| IBIS file stm32h563_573_ufbga201-smps.ibs
[IBIS ver] 4.2
[File name] stm32h563_573_ufbga201-smps.ibs
[File Rev] 1.1
[Date] 07-05-2024
[Source] Data Created at STMicroelectronics
[Notes]  File originated from ELDO simulations.
[Disclaimer]  This information is for modeling purpose only and is
   not guaranteed. The information is subject to change without
   notice.
[Copyright] Copyright 2024 STMicroelectronics Inc.
|   Component stm32h563_573_ufbga201-smps
[Component] stm32h563_573_ufbga201-smps
[Manufacturer] STMicroelectronics
[Package]
| variable   typ   min   max
R_pkg  0  NA  NA
L_pkg  0  NA  NA
C_pkg  0  NA  NA
[Pin]   signal_name   model_name
A1  PI7  io8_ft_i3c_spi
A2  PI5  io8_ft_i3c_spi
A3  VCAP  nc
A4  PB9  io8_ft_i3c_spi
A5  BOOT0  vpphv
A6  PB5  io8_ft_i3c_spi
A7  PG15  io8_ft_i3c_spi
A8  PG14  io8_ft_i3c_spi
A9  PG10  io8_ft_i3c_spi
A10  PD7  io8_ft_i3c_spi
A11  PD5  io8_ft_i3c_spi
A12  PD3  io8_ft_i3c_spi
A13  PD1  io8_ft_i3c_spi
A14  PI3  io8_ft_i3c_spi
A15  PI1  io8_ft_i3c_spi
B1  VBAT  power
B2  PE3  io8_ft_i3c_spi
B3  PI4  io8_ft_i3c_spi
B4  PE1  io8_ft_i3c_spi
B5  PB8  io8_ft_i3c_spi
B6  PB6  io8_ft_i3c_spi
B7  PB3  io8_ft_i3c_spi
B8  PG12  io8_ft_i3c_spi
B9  PG9  io8_ft_i3c_spi
B10  PD6  io8_ft_i3c_spi
B11  PD4  io8_ft_i3c_spi
B12  PD0  io8_ft_i3c_spi
B13  PA14  io8_ft_i3c_spi
B14  PI2  io8_ft_i3c_spi
B15  PH13  io8_ft_i3c_spi
C1  VSS  gnd
C2  PE6  io8_ft_i3c_spi
C3  PE4  io8_ft_i3c_spi
C4  PI6  io8_ft_i3c_spi
C5  PE0  io8_ft_i3c_spi
C6  PB7  io8_ft_i3c_spi
C7  PB4  io8_ft_i3c_spi
C8  PG13  io8_ft_i3c_spi
C9  PG11  io8_ft_i3c_spi
C10  PD2  io8_ft_i3c_spi
C11  PC12  io8_ft_i3c_spi
C12  PC11  io8_ft_i3c_spi
C13  PA15  io8_ft_i3c_spi
C14  PH15  io8_ft_i3c_spi
C15  PA12  io8usb_ft_i3c_spi_phy
D1  PC15-OSC32_OUT  io8_ft_i3c_spi
D2  PC14-OSC32_IN  io8_ft_i3c_spi
D3  PE5  io8_ft_i3c_spi
D4  PE2  io8_ft_i3c_spi
D5  VDD  power
D6  VSS  gnd
D7  VDDIO2  power
D8  VDD  power
D9  VSS  gnd
D10  VDD  power
D11  VSS  gnd
D12  PC10  io8_ft_i3c_spi
D13  PH14  io8_ft_i3c_spi
D14  VSS  gnd
D15  PA11  io8usb_ft_i3c_spi_phy
E1  PI9  io8_ft_i3c_spi
E2  PI8  io8_ft_i3c_spi
E3  PC13  io8_ft_i3c_spi
E4  VDD  power
E12  VDD  power
E13  PA13  io8_ft_i3c_spi
E14  PA10  io8_ft_i3c_spi
E15  PA9  io8_ft_i3c_spi
F1  PF1  io8_ft_i3c_spi
F2  PF0  io8_ft_i3c_spi
F3  PI11  io8_ft_i3c_spi
F4  PI10  io8_ft_i3c_spi
F6  VSS  gnd
F7  VSS  gnd
F8  VSS  gnd
F9  VSS  gnd
F10  VSS  gnd
F12  VDD33USB  power
F13  PC9  io8_ft_i3c_spi
F14  PC8  io8_ft_i3c_spi
F15  PA8  io8_ft_i3c_spi
G1  PF4  io8_ft_i3c_spi
G2  PF3  io8_ft_i3c_spi
G3  PF2  io8_ft_i3c_spi
G4  VSS  gnd
G6  VSS  gnd
G7  VSS  gnd
G8  VSS  gnd
G9  VSS  gnd
G10  VSS  gnd
G12  VSS  gnd
G13  PC7  io8_ft_i3c_spi
G14  PC6  io8_ft_i3c_spi
G15  PG8  io8_ft_i3c_spi
H1  PF6  io8_ft_i3c_spi
H2  PF8  io8_ft_i3c_spi
H3  PF5  io8_ft_i3c_spi
H4  VDD  power
H6  VSS  gnd
H7  VSS  gnd
H8  VSS  gnd
H9  VSS  gnd
H10  VSS  gnd
H12  VSS  gnd
H13  PG7  io8_ft_i3c_spi
H14  PG3  io8_ft_i3c_spi
H15  PG5  io8_ft_i3c_spi
J1  PH0-OSC_IN  io8_ft_i3c_spi
J2  PH1-OSC_OUT  io8_ft_i3c_spi
J3  PF9  io8_ft_i3c_spi
J4  PF10  io8_ft_i3c_spi
J6  VSS  gnd
J7  VSS  gnd
J8  VSS  gnd
J9  VSS  gnd
J10  VSS  gnd
J12  VDD  power
J13  PD15  io8_ft_i3c_spi
J14  PG6  io8_ft_i3c_spi
J15  PG4  io8_ft_i3c_spi
K1  VSS  gnd
K2  PF7  io8_ft_i3c_spi
K3  NRST  ioreset_ft_v33
K4  PC2  io8_ft_spi
K6  VSS  gnd
K7  VSS  gnd
K8  VSS  gnd
K9  VSS  gnd
K10  VSS  gnd
K12  PD10  io8_ft_i3c_spi
K13  PD14  io8_ft_i3c_spi
K14  PD12  io8_ft_i3c_spi
K15  PG2  io8_ft_i3c_spi
L1  PC0  io8_ft_spi
L2  PC1  io8_ft_spi
L3  PA1  io8_ft_spi_tamp
L4  VDD  power
L12  PB12  io8_ft_i3c_spi
L13  PD9  io8_ft_i3c_spi
L14  PD11  io8_ft_i3c_spi
L15  PD13  io8_ft_i3c_spi
M1  VDDA  nc
M2  VSSA  nc
M3  PA2  io8_ft_spi
M4  VSS  gnd
M5  PA4  io8_ft_spi
M6  VDD  power
M7  VSS  gnd
M8  VDD  power
M9  VSS  gnd
M10  PB10  io8_ft_i3c_spi
M11  VDD  power
M12  PH9  io8_ft_i3c_spi
M13  PH12  io8_ft_i3c_spi
M14  PB15  io8_ft_spi
M15  PD8  io8_ft_i3c_spi
N1  VREFP  nc
N2  VREFM  nc
N3  PC3  io8_ft_spi
N4  PC4  io8_ft_spi
N5  PA3  io8_ft_spi
N6  PB1  io8_ft_spi
N7  PF12  io8_ft_spi
N8  PF15  io8_ft_i3c_spi
N9  PE9  io8_ft_i3c_spi
N10  PE14  io8_ft_i3c_spi
N11  PE15  io8_ft_i3c_spi
N12  PB11  io8_ft_i3c_spi
N13  PH8  io8_ft_i3c_spi
N14  PH10  io8_ft_i3c_spi
|N15  PB14  io8usb_ft_pd
N15  PB14  nc
P1  PH5  io8_ft_i3c_spi
P2  PA0  io8_ft_spi
P3  PH3  io8_ft_i3c_spi
P4  PC5  io8_ft_spi
P5  PA6  io8_ft_spi
P6  PB2  io8_ft_i3c_spi
P7  PF13  io8_ft_spi
P8  PG1  io8_ft_i3c_spi
P9  PE8  io8_ft_i3c_spi
P10  PE11  io8_ft_i3c_spi
P11  PE13  io8_ft_i3c_spi
P12  VSSSMPS  nc
P13  PH6  io8_ft_i3c_spi
P14  PH7  io8_ft_i3c_spi
P15  PH11  io8_ft_i3c_spi
R1  PH4  io8_ft_i3c_spi
R2  PH2  io8_ft_i3c_spi
R3  PA5  io8_ft_spi
R4  PA7  io8_ft_spi
R5  PB0  io8_ft_spi
R6  PF11  io8_ft_spi
R7  PF14  io8_ft_spi
R8  PG0  io8_ft_i3c_spi
R9  PE7  io8_ft_i3c_spi
R10  PE10  io8_ft_i3c_spi
R11  PE12  io8_ft_i3c_spi
R12  VLXSMPS  nc
R13  VDDSMPS  nc
R14  VCAP  nc
|R15  PB13  io8usb_ft_pd
R15  PB13  nc
[Package Model]   484-ufbga-10x10-201-smps-221014
[Pin Mapping]   pulldown_ref   pullup_ref   | Comment
A1  gndio  vddiom
A2  gndio  vddiom
A3  nc  nc
A4  gndio  vddiom  | Depending on IO usage
| A4  gndio  vddmmc  | Depending on IO usage
A5  gndio  vddiom  | Depending on IO usage
| A5  gndio  vddmmc  | Depending on IO usage
A6  gndio  vddiom  | Depending on IO usage
| A6  gndio  vddmmc  | Depending on IO usage
A7  gndio  vddiom  | Depending on IO usage
| A7  gndio  vddmmc  | Depending on IO usage
A8  gndio  vddiom  | Depending on IO usage
| A8  gndio  vddmmc  | Depending on IO usage
A9  gndio  vddiom  | Depending on IO usage
| A9  gndio  vddmmc  | Depending on IO usage
A10  gndio  vddiom  | Depending on IO usage
| A10  gndio  vddmmc  | Depending on IO usage
A11  gndio  vddiom
A12  gndio  vddiom
A13  gndio  vddiom
A14  gndio  vddiom
A15  gndio  vddiom
B1  nc  vsw
B2  gndio  vddiom
B3  gndio  vddiom
B4  gndio  vddiom  | Depending on IO usage
| B4  gndio  vddmmc  | Depending on IO usage
B5  gndio  vddiom  | Depending on IO usage
| B5  gndio  vddmmc  | Depending on IO usage
B6  gndio  vddiom  | Depending on IO usage
| B6  gndio  vddmmc  | Depending on IO usage
B7  gndio  vddiom  | Depending on IO usage
| B7  gndio  vddmmc  | Depending on IO usage
B8  gndio  vddiom  | Depending on IO usage
| B8  gndio  vddmmc  | Depending on IO usage
B9  gndio  vddiom  | Depending on IO usage
| B9  gndio  vddmmc  | Depending on IO usage
B10  gndio  vddiom  | Depending on IO usage
| B10  gndio  vddmmc  | Depending on IO usage
B11  gndio  vddiom
B12  gndio  vddiom
B13  gndio  vddiom
B14  gndio  vddiom
B15  gndio  vddiom
C1  gndio  nc
C2  gndio  vddiom
C3  gndio  vddiom
C4  gndio  vddiom
C5  gndio  vddiom  | Depending on IO usage
| C5  gndio  vddmmc  | Depending on IO usage
C6  gndio  vddiom  | Depending on IO usage
| C6  gndio  vddmmc  | Depending on IO usage
C7  gndio  vddiom  | Depending on IO usage
| C7  gndio  vddmmc  | Depending on IO usage
C8  gndio  vddiom  | Depending on IO usage
| C8  gndio  vddmmc  | Depending on IO usage
C9  gndio  vddiom  | Depending on IO usage
| C9  gndio  vddmmc  | Depending on IO usage
C10  gndio  vddiom
C11  gndio  vddiom
C12  gndio  vddiom
C13  gndio  vddiom
C14  gndio  vddiom
C15  gndio  vddiom  | Depending on IO usage
| C15  gndio  vddusb  | Depending on IO usage
D1  gndio  vddiom  | Depending on IO usage
| D1  gndio  vsw  | Depending on IO usage
D2  gndio  vddiom  | Depending on IO usage
| D2  gndio  vsw  | Depending on IO usage
D3  gndio  vddiom
D4  gndio  vddiom
D5  nc  vddiom
D6  gndio  nc
D7  nc  vddmmc
D8  nc  vddiom
D9  gndio  nc
D10  nc  vddiom
D11  gndio  nc
D12  gndio  vddiom
D13  gndio  vddiom
D14  gndio  nc
D15  gndio  vddiom  | Depending on IO usage
| D15  gndio  vddusb  | Depending on IO usage
E1  gndio  vddiom
E2  gndio  vddiom  | Depending on IO usage
| E2  gndio  vsw  | Depending on IO usage
E3  gndio  vddiom  | Depending on IO usage
| E3  gndio  vsw  | Depending on IO usage
E4  nc  vddiom
E12  nc  vddiom
E13  gndio  vddiom  | Depending on IO usage
| E13  gndio  vddusb  | Depending on IO usage
E14  gndio  vddiom  | Depending on IO usage
| E14  gndio  vddusb  | Depending on IO usage
E15  gndio  vddiom  | Depending on IO usage
| E15  gndio  vddusb  | Depending on IO usage
F1  gndio  vddiom
F2  gndio  vddiom
F3  gndio  vddiom
F4  gndio  vddiom
F6  gndio  nc
F7  gndio  nc
F8  gndio  nc
F9  gndio  nc
F10  gndio  nc
F12  nc  vddusb
F13  gndio  vddiom
F14  gndio  vddiom
F15  gndio  vddiom
G1  gndio  vddiom
G2  gndio  vddiom
G3  gndio  vddiom
G4  gndio  nc
G6  gndio  nc
G7  gndio  nc
G8  gndio  nc
G9  gndio  nc
G10  gndio  nc
G12  gndio  nc
G13  gndio  vddiom
G14  gndio  vddiom
G15  gndio  vddiom
H1  gndio  vddiom
H2  gndio  vddiom
H3  gndio  vddiom
H4  nc  vddiom
H6  gndio  nc
H7  gndio  nc
H8  gndio  nc
H9  gndio  nc
H10  gndio  nc
H12  gndio  nc
H13  gndio  vddiom
H14  gndio  vddiom
H15  gndio  vddiom
J1  gndio  vddiom
J2  gndio  vddiom
J3  gndio  vddiom
J4  gndio  vddiom
J6  gndio  nc
J7  gndio  nc
J8  gndio  nc
J9  gndio  nc
J10  gndio  nc
J12  nc  vddiom
J13  gndio  vddiom
J14  gndio  vddiom
J15  gndio  vddiom
K1  gndio  nc
K2  gndio  vddiom
K3  gndio  vddiom
K4  gndio  vddiom
K6  gndio  nc
K7  gndio  nc
K8  gndio  nc
K9  gndio  nc
K10  gndio  nc
K12  gndio  vddiom
K13  gndio  vddiom
K14  gndio  vddiom
K15  gndio  vddiom
L1  gndio  vddiom
L2  gndio  vddiom
L3  gndio  vddiom
L4  nc  vddiom
L12  gndio  vddiom
L13  gndio  vddiom
L14  gndio  vddiom
L15  gndio  vddiom
M1  nc  nc
M2  nc  nc
M3  gndio  vddiom
M4  gndio  nc
M5  gndio  vddiom
M6  nc  vddiom
M7  gndio  nc
M8  nc  vddiom
M9  gndio  nc
M10  gndio  vddiom
M11  nc  vddiom
M12  gndio  vddiom
M13  gndio  vddiom
M14  gndio  vddiom
M15  gndio  vddiom
N1  nc  nc
N2  nc  nc
N3  gndio  vddiom
N4  gndio  vddiom
N5  gndio  vddiom
N6  gndio  vddiom
N7  gndio  vddiom
N8  gndio  vddiom
N9  gndio  vddiom
N10  gndio  vddiom
N11  gndio  vddiom
N12  gndio  vddiom
N13  gndio  vddiom
N14  gndio  vddiom
|N15  gndio  vddiom
N15  nc nc
P1  gndio  vddiom
P2  gndio  vddiom
P3  gndio  vddiom
P4  gndio  vddiom
P5  gndio  vddiom
P6  gndio  vddiom
P7  gndio  vddiom
P8  gndio  vddiom
P9  gndio  vddiom
P10  gndio  vddiom
P11  gndio  vddiom
P12  nc  nc
P13  gndio  vddiom
P14  gndio  vddiom
P15  gndio  vddiom
R1  gndio  vddiom
R2  gndio  vddiom
R3  gndio  vddiom
R4  gndio  vddiom
R5  gndio  vddiom
R6  gndio  vddiom
R7  gndio  vddiom
R8  gndio  vddiom
R9  gndio  vddiom
R10  gndio  vddiom
R11  gndio  vddiom
R12  nc  nc
R13  nc  nc
R14  nc  nc
|R15  gndio  vddiom
R15  nc nc
[Model Selector] io8_ft_i3c_spi
io8_ft_spi_ls_1v2 "io8_ft spi low speed @ 1.2V"
io8_ft_spi_ls_1v8 "io8_ft spi low speed @ 1.8V"
io8_ft_spi_ls_3v3 "io8_ft spi low speed @ 3.3V"
io8_ft_spi_ms_1v2 "io8_ft spi med speed @ 1.2V"
io8_ft_spi_ms_1v8 "io8_ft spi med speed @ 1.8V"
io8_ft_spi_ms_3v3 "io8_ft spi med speed @ 3.3V"
io8_ft_spi_fs_1v2 "io8_ft spi fast speed @ 1.2V"
io8_ft_spi_fs_1v8 "io8_ft spi fast speed @ 1.8V"
io8_ft_spi_fs_3v3 "io8_ft spi fast speed @ 3.3V"
io8_ft_spi_hs_1v2 "io8_ft spi high speed @ 1.2V"
io8_ft_spi_hs_1v8 "io8_ft spi high speed @ 1.8V"
io8_ft_spi_hs_3v3 "io8_ft spi high speed @ 3.3V"
io8_ft_hslv_spi_ls_1v2 "io8_ft spi hslv low speed @ 1.2V"
io8_ft_hslv_spi_ls_1v8 "io8_ft spi hslv low speed @ 1.8V"
io8_ft_hslv_spi_ls_2v5 "io8_ft spi hslv low speed @ 2.5V"
io8_ft_hslv_spi_ms_1v2 "io8_ft spi hslv med speed @ 1.2V"
io8_ft_hslv_spi_ms_1v8 "io8_ft spi hslv med speed @ 1.8V"
io8_ft_hslv_spi_ms_2v5 "io8_ft spi hslv med speed @ 2.5V"
io8_ft_hslv_spi_fs_1v2 "io8_ft spi hslv fast speed @ 1.2V"
io8_ft_hslv_spi_fs_1v8 "io8_ft spi hslv fast speed @ 1.8V"
io8_ft_hslv_spi_fs_2v5 "io8_ft spi hslv fast speed @ 2.5V"
io8_ft_hslv_spi_hs_1v2 "io8_ft spi hslv high speed @ 1.2V"
io8_ft_hslv_spi_hs_1v8 "io8_ft spi hslv high speed @ 1.8V"
io8_ft_hslv_spi_hs_2v5 "io8_ft spi hslv high speed @ 2.5V"
io8_ft_i3c_spi_ls_1v2 "io8_ft i3c spi open-drain low speed @ 1.2V"
io8_ft_i3c_spi_ls_1v8 "io8_ft i3c spi open-drain low speed @ 1.8V"
io8_ft_i3c_spi_ls_3v3 "io8_ft i3c spi open-drain low speed @ 3.3V"
io8_ft_i3c_spi_ms_1v2 "io8_ft i3c spi open-drain med speed @ 1.2V"
io8_ft_i3c_spi_ms_1v8 "io8_ft i3c spi open-drain med speed @ 1.8V"
io8_ft_i3c_spi_ms_3v3 "io8_ft i3c spi open-drain med speed @ 3.3V"
io8_ft_i3c_spi_fs_1v2 "io8_ft i3c spi open-drain fast speed @ 1.2V"
io8_ft_i3c_spi_fs_1v8 "io8_ft i3c spi open-drain fast speed @ 1.8V"
io8_ft_i3c_spi_fs_3v3 "io8_ft i3c spi open-drain fast speed @ 3.3V"
io8_ft_i3c_spi_hs_1v2 "io8_ft i3c spi open-drain high speed @ 1.2V"
io8_ft_i3c_spi_hs_1v8 "io8_ft i3c spi open-drain high speed @ 1.8V"
io8_ft_i3c_spi_hs_3v3 "io8_ft i3c spi open-drain high speed @ 3.3V"
io8_ft_hslv_i3c_spi_ls_1v2 "io8_ft hslv i3c spi open-drain low speed @ 1.2V"
io8_ft_hslv_i3c_spi_ls_1v8 "io8_ft hslv i3c spi open-drain low speed @ 1.8V"
io8_ft_hslv_i3c_spi_ls_2v5 "io8_ft hslv i3c spi open-drain low speed @ 2.5V"
io8_ft_hslv_i3c_spi_ms_1v2 "io8_ft hslv i3c spi open-drain med speed @ 1.2V"
io8_ft_hslv_i3c_spi_ms_1v8 "io8_ft hslv i3c spi open-drain med speed @ 1.8V"
io8_ft_hslv_i3c_spi_ms_2v5 "io8_ft hslv i3c spi open-drain med speed @ 2.5V"
io8_ft_hslv_i3c_spi_fs_1v2 "io8_ft hslv i3c spi open-drain fast speed @ 1.2V"
io8_ft_hslv_i3c_spi_fs_1v8 "io8_ft hslv i3c spi open-drain fast speed @ 1.8V"
io8_ft_hslv_i3c_spi_fs_2v5 "io8_ft hslv i3c spi open-drain fast speed @ 2.5V"
io8_ft_hslv_i3c_spi_hs_1v2 "io8_ft hslv i3c spi open-drain high speed @ 1.2V"
io8_ft_hslv_i3c_spi_hs_1v8 "io8_ft hslv i3c spi open-drain high speed @ 1.8V"
io8_ft_hslv_i3c_spi_hs_2v5 "io8_ft hslv i3c spi open-drain high speed @ 2.5V"
io8_ft_i3c_fmp_spi_3v3 "io8_ft i3c fm+ spi open-drain @ 3.3V"
io8_ft_i3c_fmp_spi_1v8 "io8_ft i3c fm+ spi open-drain @ 1.8V"
io8_ft_i3c_fmp_spi_1v2 "io8_ft i3c fm+ spi open-drain @ 1.2V"
[Model Selector] io8_ft_spi
io8_ft_spi_ls_1v2 "io8_ft spi low speed @ 1.2V"
io8_ft_spi_ls_1v8 "io8_ft spi low speed @ 1.8V"
io8_ft_spi_ls_3v3 "io8_ft spi low speed @ 3.3V"
io8_ft_spi_ms_1v2 "io8_ft spi med speed @ 1.2V"
io8_ft_spi_ms_1v8 "io8_ft spi med speed @ 1.8V"
io8_ft_spi_ms_3v3 "io8_ft spi med speed @ 3.3V"
io8_ft_spi_fs_1v2 "io8_ft spi fast speed @ 1.2V"
io8_ft_spi_fs_1v8 "io8_ft spi fast speed @ 1.8V"
io8_ft_spi_fs_3v3 "io8_ft spi fast speed @ 3.3V"
io8_ft_spi_hs_1v2 "io8_ft spi high speed @ 1.2V"
io8_ft_spi_hs_1v8 "io8_ft spi high speed @ 1.8V"
io8_ft_spi_hs_3v3 "io8_ft spi high speed @ 3.3V"
io8_ft_hslv_spi_ls_1v2 "io8_ft spi hslv low speed @ 1.2V"
io8_ft_hslv_spi_ls_1v8 "io8_ft spi hslv low speed @ 1.8V"
io8_ft_hslv_spi_ls_2v5 "io8_ft spi hslv low speed @ 2.5V"
io8_ft_hslv_spi_ms_1v2 "io8_ft spi hslv med speed @ 1.2V"
io8_ft_hslv_spi_ms_1v8 "io8_ft spi hslv med speed @ 1.8V"
io8_ft_hslv_spi_ms_2v5 "io8_ft spi hslv med speed @ 2.5V"
io8_ft_hslv_spi_fs_1v2 "io8_ft spi hslv fast speed @ 1.2V"
io8_ft_hslv_spi_fs_1v8 "io8_ft spi hslv fast speed @ 1.8V"
io8_ft_hslv_spi_fs_2v5 "io8_ft spi hslv fast speed @ 2.5V"
io8_ft_hslv_spi_hs_1v2 "io8_ft spi hslv high speed @ 1.2V"
io8_ft_hslv_spi_hs_1v8 "io8_ft spi hslv high speed @ 1.8V"
io8_ft_hslv_spi_hs_2v5 "io8_ft spi hslv high speed @ 2.5V"
[Model Selector] io8_ft_spi_tamp
io8_ft_spi_ls_1v2 "io8_ft spi low speed @ 1.2V"
io8_ft_spi_ls_1v8 "io8_ft spi low speed @ 1.8V"
io8_ft_spi_ls_3v3 "io8_ft spi low speed @ 3.3V"
io8_ft_spi_ms_1v2 "io8_ft spi med speed @ 1.2V"
io8_ft_spi_ms_1v8 "io8_ft spi med speed @ 1.8V"
io8_ft_spi_ms_3v3 "io8_ft spi med speed @ 3.3V"
io8_ft_spi_fs_1v2 "io8_ft spi fast speed @ 1.2V"
io8_ft_spi_fs_1v8 "io8_ft spi fast speed @ 1.8V"
io8_ft_spi_fs_3v3 "io8_ft spi fast speed @ 3.3V"
io8_ft_spi_hs_1v2 "io8_ft spi high speed @ 1.2V"
io8_ft_spi_hs_1v8 "io8_ft spi high speed @ 1.8V"
io8_ft_spi_hs_3v3 "io8_ft spi high speed @ 3.3V"
io8_ft_hslv_spi_ls_1v2 "io8_ft spi hslv low speed @ 1.2V"
io8_ft_hslv_spi_ls_1v8 "io8_ft spi hslv low speed @ 1.8V"
io8_ft_hslv_spi_ls_2v5 "io8_ft spi hslv low speed @ 2.5V"
io8_ft_hslv_spi_ms_1v2 "io8_ft spi hslv med speed @ 1.2V"
io8_ft_hslv_spi_ms_1v8 "io8_ft spi hslv med speed @ 1.8V"
io8_ft_hslv_spi_ms_2v5 "io8_ft spi hslv med speed @ 2.5V"
io8_ft_hslv_spi_fs_1v2 "io8_ft spi hslv fast speed @ 1.2V"
io8_ft_hslv_spi_fs_1v8 "io8_ft spi hslv fast speed @ 1.8V"
io8_ft_hslv_spi_fs_2v5 "io8_ft spi hslv fast speed @ 2.5V"
io8_ft_hslv_spi_hs_1v2 "io8_ft spi hslv high speed @ 1.2V"
io8_ft_hslv_spi_hs_1v8 "io8_ft spi hslv high speed @ 1.8V"
io8_ft_hslv_spi_hs_2v5 "io8_ft spi hslv high speed @ 2.5V"
io8_ft_tamp_v33_1v2 "io8_ft tamp V33 @ 1.2V"
io8_ft_tamp_v33_1v8 "io8_ft tamp V33 @ 1.2V"
io8_ft_tamp_v33_3v3 "io8_ft tamp V33 @ 1.2V"
[Model Selector] io8usb_ft_i3c_spi_phy
io8_ft_spi_ls_1v2 "io8_ft spi low speed @ 1.2V"
io8_ft_spi_ls_1v8 "io8_ft spi low speed @ 1.8V"
io8_ft_spi_ls_3v3 "io8_ft spi low speed @ 3.3V"
io8_ft_spi_ms_1v2 "io8_ft spi med speed @ 1.2V"
io8_ft_spi_ms_1v8 "io8_ft spi med speed @ 1.8V"
io8_ft_spi_ms_3v3 "io8_ft spi med speed @ 3.3V"
io8_ft_spi_fs_1v2 "io8_ft spi fast speed @ 1.2V"
io8_ft_spi_fs_1v8 "io8_ft spi fast speed @ 1.8V"
io8_ft_spi_fs_3v3 "io8_ft spi fast speed @ 3.3V"
io8_ft_spi_hs_1v2 "io8_ft spi high speed @ 1.2V"
io8_ft_spi_hs_1v8 "io8_ft spi high speed @ 1.8V"
io8_ft_spi_hs_3v3 "io8_ft spi high speed @ 3.3V"
io8_ft_hslv_spi_ls_1v2 "io8_ft spi hslv low speed @ 1.2V"
io8_ft_hslv_spi_ls_1v8 "io8_ft spi hslv low speed @ 1.8V"
io8_ft_hslv_spi_ls_2v5 "io8_ft spi hslv low speed @ 2.5V"
io8_ft_hslv_spi_ms_1v2 "io8_ft spi hslv med speed @ 1.2V"
io8_ft_hslv_spi_ms_1v8 "io8_ft spi hslv med speed @ 1.8V"
io8_ft_hslv_spi_ms_2v5 "io8_ft spi hslv med speed @ 2.5V"
io8_ft_hslv_spi_fs_1v2 "io8_ft spi hslv fast speed @ 1.2V"
io8_ft_hslv_spi_fs_1v8 "io8_ft spi hslv fast speed @ 1.8V"
io8_ft_hslv_spi_fs_2v5 "io8_ft spi hslv fast speed @ 2.5V"
io8_ft_hslv_spi_hs_1v2 "io8_ft spi hslv high speed @ 1.2V"
io8_ft_hslv_spi_hs_1v8 "io8_ft spi hslv high speed @ 1.8V"
io8_ft_hslv_spi_hs_2v5 "io8_ft spi hslv high speed @ 2.5V"
io8_ft_i3c_spi_ls_1v2 "io8_ft i3c spi open-drain low speed @ 1.2V"
io8_ft_i3c_spi_ls_1v8 "io8_ft i3c spi open-drain low speed @ 1.8V"
io8_ft_i3c_spi_ls_3v3 "io8_ft i3c spi open-drain low speed @ 3.3V"
io8_ft_i3c_spi_ms_1v2 "io8_ft i3c spi open-drain med speed @ 1.2V"
io8_ft_i3c_spi_ms_1v8 "io8_ft i3c spi open-drain med speed @ 1.8V"
io8_ft_i3c_spi_ms_3v3 "io8_ft i3c spi open-drain med speed @ 3.3V"
io8_ft_i3c_spi_fs_1v2 "io8_ft i3c spi open-drain fast speed @ 1.2V"
io8_ft_i3c_spi_fs_1v8 "io8_ft i3c spi open-drain fast speed @ 1.8V"
io8_ft_i3c_spi_fs_3v3 "io8_ft i3c spi open-drain fast speed @ 3.3V"
io8_ft_i3c_spi_hs_1v2 "io8_ft i3c spi open-drain high speed @ 1.2V"
io8_ft_i3c_spi_hs_1v8 "io8_ft i3c spi open-drain high speed @ 1.8V"
io8_ft_i3c_spi_hs_3v3 "io8_ft i3c spi open-drain high speed @ 3.3V"
io8_ft_hslv_i3c_spi_ls_1v2 "io8_ft hslv i3c spi open-drain low speed @ 1.2V"
io8_ft_hslv_i3c_spi_ls_1v8 "io8_ft hslv i3c spi open-drain low speed @ 1.8V"
io8_ft_hslv_i3c_spi_ls_2v5 "io8_ft hslv i3c spi open-drain low speed @ 2.5V"
io8_ft_hslv_i3c_spi_ms_1v2 "io8_ft hslv i3c spi open-drain med speed @ 1.2V"
io8_ft_hslv_i3c_spi_ms_1v8 "io8_ft hslv i3c spi open-drain med speed @ 1.8V"
io8_ft_hslv_i3c_spi_ms_2v5 "io8_ft hslv i3c spi open-drain med speed @ 2.5V"
io8_ft_hslv_i3c_spi_fs_1v2 "io8_ft hslv i3c spi open-drain fast speed @ 1.2V"
io8_ft_hslv_i3c_spi_fs_1v8 "io8_ft hslv i3c spi open-drain fast speed @ 1.8V"
io8_ft_hslv_i3c_spi_fs_2v5 "io8_ft hslv i3c spi open-drain fast speed @ 2.5V"
io8_ft_hslv_i3c_spi_hs_1v2 "io8_ft hslv i3c spi open-drain high speed @ 1.2V"
io8_ft_hslv_i3c_spi_hs_1v8 "io8_ft hslv i3c spi open-drain high speed @ 1.8V"
io8_ft_hslv_i3c_spi_hs_2v5 "io8_ft hslv i3c spi open-drain high speed @ 2.5V"
io8_ft_i3c_fmp_spi_3v3 "io8_ft i3c fm+ spi open-drain @ 3.3V"
io8_ft_i3c_fmp_spi_1v8 "io8_ft i3c fm+ spi open-drain @ 1.8V"
io8_ft_i3c_fmp_spi_1v2 "io8_ft i3c fm+ spi open-drain @ 1.2V"
io8usb_ft_phy_ls_2v5 "iousb ft low speed @ 2.5V"
io8usb_ft_phy_ls_3v3 "iousb ft low speed @ 3.3V"
io8usb_ft_phy_fs_2v5 "iousb ft fast speed @ 2.5V"
io8usb_ft_phy_fs_3v3 "iousb ft fast speed @ 3.3V"
[Model Selector] ioreset_ft_v33
ioreset_ft_v33_1v2 "Reset PAD. 5V tolerant. 1.2V range"
ioreset_ft_v33_1v8 "Reset PAD. 5V tolerant. 1.8V range"
ioreset_ft_v33_3v3 "Reset PAD. 5V tolerant. 3.3V range"
[Model Selector] vpphv
vpphv_1v2 "Flash Test cell v33 = 1.2 V range"
vpphv_1v8 "Flash Test cell v33 = 1.8 V range"
vpphv_3v3 "Flash Test cell v33 = 3.3 V range"
[Define Package Model]  484-ufbga-10x10-201-smps-221014
[Manufacturer]  unknown
[OEM]  unknown
[Description]  unknown
[Number Of Pins]  155
[Pin Numbers]
| Pin Name Terminal   Net Name   Starting Node   Ending Node
A5 | BOOT0
K3 | NRST
P2 | PA0
L3 | PA1
M3 | PA2
N5 | PA3
M5 | PA4
R3 | PA5
P5 | PA6
R4 | PA7
F15 | PA8
E15 | PA9
E14 | PA10
D15 | PA11
C15 | PA12
E13 | PA13
B13 | PA14
C13 | PA15
R5 | PB0
N6 | PB1
P6 | PB2
B7 | PB3
C7 | PB4
A6 | PB5
B6 | PB6
C6 | PB7
B5 | PB8
A4 | PB9
M10 | PB10
N12 | PB11
L12 | PB12
R15 | PB13
N15 | PB14
M14 | PB15
L1 | PC0
L2 | PC1
K4 | PC2
N3 | PC3
N4 | PC4
P4 | PC5
G14 | PC6
G13 | PC7
F14 | PC8
F13 | PC9
D12 | PC10
C12 | PC11
C11 | PC12
E3 | PC13
D2 | PC14-OSC32_IN
D1 | PC15-OSC32_OUT
B12 | PD0
A13 | PD1
C10 | PD2
A12 | PD3
B11 | PD4
A11 | PD5
B10 | PD6
A10 | PD7
M15 | PD8
L13 | PD9
K12 | PD10
L14 | PD11
K14 | PD12
L15 | PD13
K13 | PD14
J13 | PD15
C5 | PE0
B4 | PE1
D4 | PE2
B2 | PE3
C3 | PE4
D3 | PE5
C2 | PE6
R9 | PE7
P9 | PE8
N9 | PE9
R10 | PE10
P10 | PE11
R11 | PE12
P11 | PE13
N10 | PE14
N11 | PE15
F2 | PF0
F1 | PF1
G3 | PF2
G2 | PF3
G1 | PF4
H3 | PF5
H1 | PF6
K2 | PF7
H2 | PF8
J3 | PF9
J4 | PF10
R6 | PF11
N7 | PF12
P7 | PF13
R7 | PF14
N8 | PF15
R8 | PG0
P8 | PG1
K15 | PG2
H14 | PG3
J15 | PG4
H15 | PG5
J14 | PG6
H13 | PG7
G15 | PG8
B9 | PG9
A9 | PG10
C9 | PG11
B8 | PG12
C8 | PG13
A8 | PG14
A7 | PG15
J1 | PH0-OSC_IN
J2 | PH1-OSC_OUT
R2 | PH2
P3 | PH3
R1 | PH4
P1 | PH5
P13 | PH6
P14 | PH7
N13 | PH8
M12 | PH9
N14 | PH10
P15 | PH11
M13 | PH12
B15 | PH13
D13 | PH14
C14 | PH15
A15 | PI1
B14 | PI2
A14 | PI3
B3 | PI4
A2 | PI5
C4 | PI6
A1 | PI7
E2 | PI8
E1 | PI9
F4 | PI10
F3 | PI11
B1 | VBAT
R14 | VCAP
A3 | VCAP
F12 | VDD33USB
D5 | VDD
M1 | VDDA
R13 | VDDSMPS
D7 | VDDIO2
R12 | VLXSMPS
N2 | VREFM
N1 | VREFP
C1 | VSS
M2 | VSSA
P12 | VSSSMPS
|[Merged Pins]  D5
|D8  |  VDD
|D10  |  VDD
|E4  |  VDD
|E12  |  VDD
|H4  |  VDD
|J12  |  VDD
|L4  |  VDD
|M6  |  VDD
|M8  |  VDD
|M11  |  VDD
|[Merged Pins]  C1
|D6  |  VSS
|D9  |  VSS
|D11  |  VSS
|D14  |  VSS
|F6  |  VSS
|F7  |  VSS
|F8  |  VSS
|F9  |  VSS
|F10  |  VSS
|G4  |  VSS
|G6  |  VSS
|G7  |  VSS
|G8  |  VSS
|G9  |  VSS
|G10  |  VSS
|G12  |  VSS
|H6  |  VSS
|H7  |  VSS
|H8  |  VSS
|H9  |  VSS
|H10  |  VSS
|H12  |  VSS
|J6  |  VSS
|J7  |  VSS
|J8  |  VSS
|J9  |  VSS
|J10  |  VSS
|K1  |  VSS
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[Model Data]
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[End Model Data]
[End Package Model]
|End [Component]
| Models and submodels in the file (64): io8_ft_hslv_i3c_spi_fs_1v2 (I/O_open_drain), io8_ft_hslv_i3c_spi_fs_1v8 (I/O_open_drain), io8_ft_hslv_i3c_spi_fs_2v5 (I/O_open_drain), io8_ft_hslv_i3c_spi_hs_1v2 (I/O_open_drain), io8_ft_hslv_i3c_spi_hs_1v8 (I/O_open_drain), io8_ft_hslv_i3c_spi_hs_2v5 (I/O_open_drain), io8_ft_hslv_i3c_spi_ls_1v2 (I/O_open_drain), io8_ft_hslv_i3c_spi_ls_1v8 (I/O_open_drain), io8_ft_hslv_i3c_spi_ls_2v5 (I/O_open_drain), io8_ft_hslv_i3c_spi_ms_1v2 (I/O_open_drain), io8_ft_hslv_i3c_spi_ms_1v8 (I/O_open_drain), io8_ft_hslv_i3c_spi_ms_2v5 (I/O_open_drain), io8_ft_hslv_spi_fs_1v2 (I/O), io8_ft_hslv_spi_fs_1v8 (I/O), io8_ft_hslv_spi_fs_2v5 (I/O), io8_ft_hslv_spi_hs_1v2 (I/O), io8_ft_hslv_spi_hs_1v8 (I/O), io8_ft_hslv_spi_hs_2v5 (I/O), io8_ft_hslv_spi_ls_1v2 (I/O), io8_ft_hslv_spi_ls_1v8 (I/O), io8_ft_hslv_spi_ls_2v5 (I/O), io8_ft_hslv_spi_ms_1v2 (I/O), io8_ft_hslv_spi_ms_1v8 (I/O), io8_ft_hslv_spi_ms_2v5 (I/O), io8_ft_i3c_fmp_spi_1v2 (I/O_open_drain), io8_ft_i3c_fmp_spi_1v8 (I/O_open_drain), io8_ft_i3c_fmp_spi_3v3 (I/O_open_drain), io8_ft_i3c_spi_fs_1v2 (I/O_open_drain), io8_ft_i3c_spi_fs_1v8 (I/O_open_drain), io8_ft_i3c_spi_fs_3v3 (I/O_open_drain), io8_ft_i3c_spi_hs_1v2 (I/O_open_drain), io8_ft_i3c_spi_hs_1v8 (I/O_open_drain), io8_ft_i3c_spi_hs_3v3 (I/O_open_drain), io8_ft_i3c_spi_ls_1v2 (I/O_open_drain), io8_ft_i3c_spi_ls_1v8 (I/O_open_drain), io8_ft_i3c_spi_ls_3v3 (I/O_open_drain), io8_ft_i3c_spi_ms_1v2 (I/O_open_drain), io8_ft_i3c_spi_ms_1v8 (I/O_open_drain), io8_ft_i3c_spi_ms_3v3 (I/O_open_drain), io8_ft_spi_fs_1v2 (I/O), io8_ft_spi_fs_1v8 (I/O), io8_ft_spi_fs_3v3 (I/O), io8_ft_spi_hs_1v2 (I/O), io8_ft_spi_hs_1v8 (I/O), io8_ft_spi_hs_3v3 (I/O), io8_ft_spi_ls_1v2 (I/O), io8_ft_spi_ls_1v8 (I/O), io8_ft_spi_ls_3v3 (I/O), io8_ft_spi_ms_1v2 (I/O), io8_ft_spi_ms_1v8 (I/O), io8_ft_spi_ms_3v3 (I/O), io8_ft_tamp_v33_1v2 (I/O), io8_ft_tamp_v33_1v8 (I/O), io8_ft_tamp_v33_3v3 (I/O), io8usb_ft_phy_fs_2v5 (I/O), io8usb_ft_phy_fs_3v3 (I/O), io8usb_ft_phy_ls_2v5 (I/O), io8usb_ft_phy_ls_3v3 (I/O), ioreset_ft_v33_1v2 (I/O_open_drain), ioreset_ft_v33_1v8 (I/O_open_drain), ioreset_ft_v33_3v3 (I/O_open_drain), vpphv_1v2 (Input), vpphv_1v8 (Input), vpphv_3v3 (Input)
